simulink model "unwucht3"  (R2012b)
settings: Solver=ode45  StartTime=0.0  StopTime=10.0  RelTol=1e-3
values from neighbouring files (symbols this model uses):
  a1T = a1T{:}    [unwucht_2.m]    (also in unwucht_3.m; unwucht_4.m; unwucht_5.m)
  a2T = a2T{:}    [unwucht_2.m]    (also in unwucht_3.m; unwucht_4.m; unwucht_5.m)
  b1T = b1T{:}    [unwucht_2.m]    (also in unwucht_3.m; unwucht_4.m; unwucht_5.m)
  b2T = b2T{:}    [unwucht_2.m]    (also in unwucht_3.m; unwucht_4.m; unwucht_5.m)
  m0 = 1    [unwucht_1.m]    (also in unwucht_2.m; unwucht_3.m; unwucht_4.m; unwucht_5.m)
  omega = xy.signals.values(:,2)    [gleichstrom_motor_1.m]    (also in unwucht_1.m = (2*pi)*f; unwucht_2.m = omega_0; unwucht_3.m = omega_0; unwucht_rueckw_1.m = omega(nsta:end))

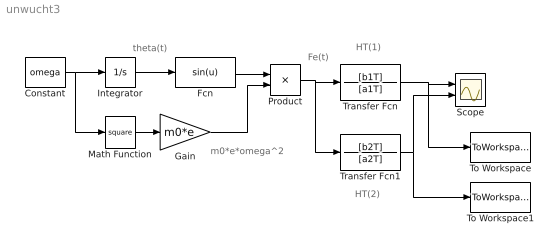
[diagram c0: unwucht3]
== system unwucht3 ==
  note: m0*e*omega^2
  note: theta(t)
  note: Fe(t)
  note: HT(2)
  note: HT(1)
  Constant : Constant  Value=omega
  Fcn : Fcn  Expr=sin(u)
  Gain : Gain  Gain=m0*e
  Integrator : Integrator
  Math Function : Math  Operator=square
  Product : Product
  Scope : Scope  NumInputPorts=2
  To Workspace : ToWorkspace  VariableName=x  SampleTime=-1  SaveFormat=Structure With Time
  To Workspace1 : ToWorkspace  VariableName=xT  SampleTime=-1  SaveFormat=Structure With Time
  Transfer Fcn : TransferFcn  Numerator=[b1T]  Denominator=[a1T]
  Transfer Fcn1 : TransferFcn  Numerator=[b2T]  Denominator=[a2T]
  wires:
  Constant/1 -> Math Function/1, Integrator/1
  Math Function/1 -> Gain/1
  Integrator/1 -> Fcn/1
  Fcn/1 -> Product/1
  Gain/1 -> Product/2
  Product/1 -> Transfer Fcn1/1, Transfer Fcn/1
  Transfer Fcn/1 -> To Workspace/1, Scope/1
  Transfer Fcn1/1 -> To Workspace1/1, Scope/2
